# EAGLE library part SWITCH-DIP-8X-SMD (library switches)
8 x SPST Dip Switch Digi-Key Part Number 1-1825058-9-ND
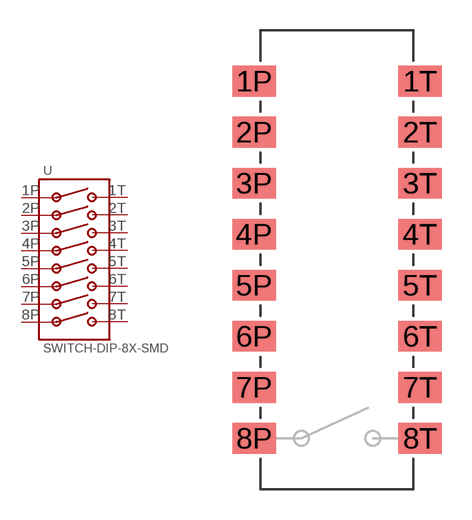
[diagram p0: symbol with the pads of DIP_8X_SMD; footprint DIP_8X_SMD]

Designator prefix -

## SWITCH-DIP-8X-SMD (DIGIKEY: 1-1825058-9-ND)  [DIP_8X_SMD]
1P  1P
1T  1T
2P  2P
2T  2T
3P  3P
3T  3T
4P  4P
4T  4T
5P  5P
5T  5T
6P  6P
6T  6T
7P  7P
7T  7T
8P  8P
8T  8T

## Footprint DIP_8X_SMD (pad centres in mm)
smd 2.159 x 1.524: 1P -4.128,8.89; 1T 4.128,8.89; 2P -4.128,6.35; 2T 4.128,6.35; 3P -4.128,3.81; 3T 4.128,3.81; 4P -4.128,1.27; 4T 4.128,1.27; 5P -4.128,-1.27; 5T 4.128,-1.27; 6P -4.128,-3.81; 6T 4.128,-3.81; 7P -4.128,-6.35; 7T 4.128,-6.35; 8P -4.128,-8.89; 8T 4.128,-8.89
